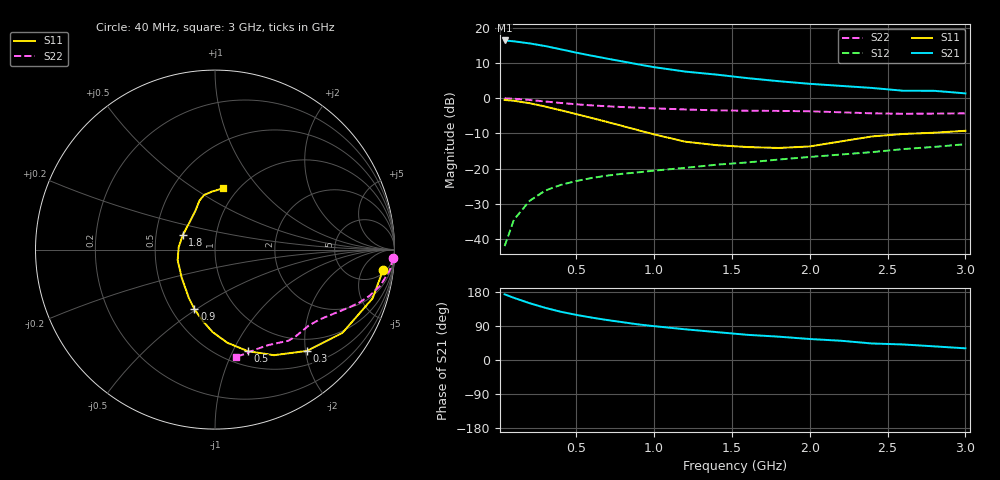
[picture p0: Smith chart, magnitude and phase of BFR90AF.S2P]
! Filename:  BFR90AF.S2P  Version:  2.0
! Philips part #: BFR90A  Date: Jul 1990
! Bias condition: Vce=10V, Ic=2mA
#  MHz  S  MA  R  50
! Freq  S11  S21  S12  S22  !GUM [dB]
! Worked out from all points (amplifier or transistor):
!   21 points, 40 MHz to 3 GHz, reference 50 ohm
!   highest |S21| = 16.4 dB at 40 MHz (marker M1)
!   |S21| within 3 dB of that: start of sweep to 452.6 MHz
!   unconditionally stable (mu >= 1): 1.19 GHz to end of sweep
!   at 300 MHz: K = 0.30, MSG = 20.5 dB, |S12| = -26.2 dB
!   at 1 GHz: K = 0.88, MSG = 14.7 dB, |S12| = -20.5 dB
!   at 3 GHz: K = 1.21, MAG = 4.5 dB, |S12| = -13.0 dB
!   S11 on the Smith chart (normalised r, x): 40 MHz: 6, -13; 300 MHz: 0.75, -2.03; 500 MHz: 0.65, -1.14; 900 MHz: 0.65, -0.49; 1.8 GHz: 0.69, +0.12; 3 GHz: 0.86, +0.67
40  0.943 -7.0  6.572 173.3  0.008 86.0  0.994 -2.7
100  0.919 -17.2  6.389 164.0  0.019 80.5  0.982 -6.5
200  0.848 -33.2  5.972 150.0  0.035 72.4  0.944 -12.2
300  0.762 -47.8  5.479 137.8  0.049 66.2  0.898 -16.7
400  0.674 -60.8  4.929 127.4  0.059 61.8  0.856 -20.2
500  0.594 -72.2  4.417 119.1  0.067 59.2  0.819 -22.9
600  0.523 -82.5  3.996 111.8  0.074 57.5  0.79 -25.1
700  0.46 -91.6  3.629 105.4  0.08 56.4  0.767 -27.0
800  0.402 -100.0  3.307 99.6  0.085 56.0  0.748 -28.7
900  0.351 -109.0  3.011 93.9  0.089 56.0  0.733 -30.2
1000  0.307 -118.3  2.751 89.3  0.094 56.3  0.718 -31.7
1200  0.242 -140.3  2.381 81.0  0.103 57.5  0.692 -35.2
1400  0.216 -164.3  2.158 73.7  0.114 58.0  0.672 -39.1
1600  0.203 176.2  1.922 66.4  0.123 60.4  0.664 -43.3
1800  0.197 155.9  1.741 61.6  0.135 61.8  0.66 -47.3
2000  0.207 133.6  1.597 55.4  0.147 62.9  0.652 -51.1
2200  0.244 116.3  1.493 50.8  0.159 63.5  0.631 -55.2
2400  0.287 107.5  1.396 43.6  0.172 64.6  0.61 -60.6
2600  0.311 101.0  1.274 41.0  0.19 64.5  0.601 -67.3
2800  0.324 92.7  1.271 36.0  0.204 64.6  0.605 -73.9
3000  0.345 82.3  1.169 30.8  0.223 65.7  0.609 -79.1
